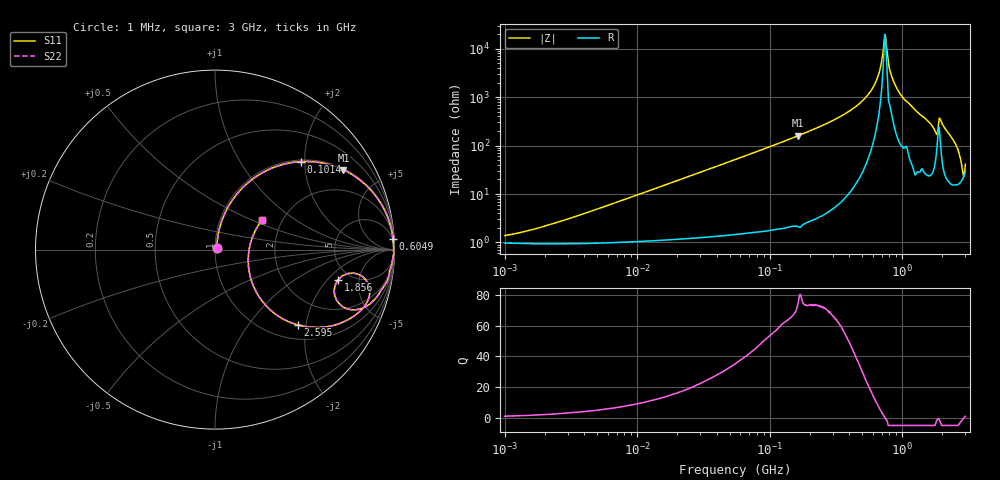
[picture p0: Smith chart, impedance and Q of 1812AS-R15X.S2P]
!s-Parameter Generated by FASTRON Sdn. Bhd.
!FASTRON P/N : 1812AS-R15X
!Keysight Technologies,E4991B,MY54100416,A.01.15
!Date created: Fri Oct 13 14:55:18 2023
!Version  : Rev00 Fri Oct 13 14:55:18 2023
!Data & Calibration Information:
!Freq	S11	S21	S12	S22
!PortZ  Port1:50+j0  Port2:50+j0
!When reading, reference impedance value at option line is always used.
! Remarks : This data is being provided solely for informational purposes.
# Hz S dB R 50
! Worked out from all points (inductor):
!   1601 points, 1 MHz to 3 GHz, reference 50 ohm
!   read as one part in series: L = 154 nH near 2.918 MHz
!   highest Q = 74.8 at 164.7 MHz (marker M1), where L = 154 nH
!   self-resonance near 742.7 MHz
!   S11 on the Smith chart (normalised r, x): 1 MHz: 1.02, +0.02; 101.4 MHz: 1.04, +1.91; 604.9 MHz: 3, +32; 1.856 GHz: 3.96, -2.64; 2.595 GHz: 1.31, -1.80; 3 GHz: 1.58, +0.58
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1000000  -37.26 44.7  -0.08 -0.6  -0.08 -0.6  -37.26 44.7
3804036  -28.52 73.4  -0.09 -2.1  -0.09 -2.1  -28.52 73.4
1.447069e7  -17.45 77.7  -0.17 -7.7  -0.17 -7.7  -17.45 77.7
5.477226e7  -6.92 61.6  -1.11 -26.8  -1.11 -26.8  -6.92 61.6
1.013595e8  -3.29 45.7  -2.90 -43.2  -2.90 -43.2  -3.29 45.7
1.646891e8  -1.49 31.8  -5.56 -57.4  -5.56 -57.4  -1.49 31.8
2.083556e8  -0.94 25.5  -7.33 -63.7  -7.33 -63.7  -0.94 25.5
4.156301e8  -0.17 10.2  -15.02 -78.5  -15.02 -78.5  -0.17 10.2
6.049187e8  -0.05 3.5  -24.22 -82.4  -24.22 -82.4  -0.05 3.5
6.719458e8  -0.04 1.7  -30.38 -79.3  -30.38 -79.3  -0.04 1.7
7.352784e8  -0.04 0.2  -44.63 -30.5  -44.63 -30.5  -0.04 0.2
7.576891e8  -0.04 -0.3  -42.22 48.8  -42.22 48.8  -0.04 -0.3
7.925923e8  -0.03 -1.2  -33.41 78.9  -33.41 78.9  -0.03 -1.2
8.629671e8  -0.07 -2.7  -26.44 79.5  -26.44 79.5  -0.07 -2.7
1.017911e9  -0.13 -5.9  -19.76 78.7  -19.76 78.7  -0.13 -5.9
1.75626e9  -1.44 -23.3  -7.90 56.5  -7.90 56.5  -1.44 -23.3
1.855641e9  -3.02 -13.7  -8.97 28.1  -8.97 28.1  -3.02 -13.7
1.950859e9  -1.00 -14.7  -11.55 58.6  -11.55 58.6  -1.00 -14.7
2.061253e9  -1.02 -21.1  -8.82 62.0  -8.82 62.0  -1.02 -21.1
2.594767e9  -4.11 -42.3  -3.31 37.9  -3.31 37.9  -4.11 -42.3
2.853575e9  -12.11 -37.6  -1.75 10.7  -1.75 10.7  -12.11 -37.6
3e9  -10.16 32.2  -2.43 -12.7  -2.43 -12.7  -10.16 32.2
